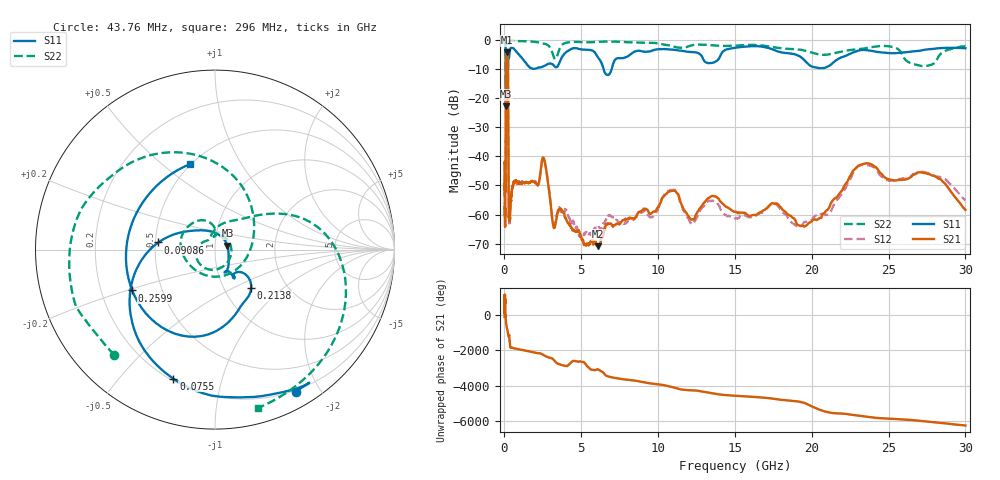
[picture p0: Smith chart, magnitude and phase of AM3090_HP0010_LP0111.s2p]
! Date/Time: Thu, Feb 28, 2019 1:55 PM
! Network Analyzer: Agilent Technologies E8364B Rev: A.07.50.67
! Sweep from 0.010 to 30.000 GHz, 1601 Points, Sweep Type: LOG
! Power Supply: 5.023 V, 0.002 A
# Hz S DB R 50
!freq MagS11 AngS11 MagS21 AngS21 MagS12 AngS12 MagS22 AngS22
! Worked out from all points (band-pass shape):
!   1601 points, 10 MHz to 30 GHz, reference 50 ohm
!   highest |S21| = -4.23 dB at 147.6 MHz (marker M1); lowest = -70.9 dB at 6.08 GHz (marker M2)
!   |S21| within 3 dB of the highest: 101.6 MHz to 216.8 MHz (115.2 MHz wide, 72.4 % of centre)
!   lowest |S11| = -22.8 dB at 99.43 MHz (marker M3), VSWR 1.16, Z = 57.4 + j2.54 ohm
!   |S11| at or under -10 dB: 90.9 MHz to 217.7 MHz (126.8 MHz wide, 82.2 % of centre); 6.451 GHz to 6.979 GHz (528.7 MHz wide, 7.87 % of centre)
!   |S22| runs from -23.8 to -0.2 dB; largest |S21 - S12| = 0.014
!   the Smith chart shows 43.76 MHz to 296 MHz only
!   S11 on the Smith chart (normalised r, x): 43.76 MHz: 0.18, -1.71; 75.5 MHz: 0.21, -0.71; 90.86 MHz: 0.52, +0.05; 213.8 MHz: 1.33, -0.63; 259.9 MHz: 0.34, -0.21; 296 MHz: 0.49, +0.62
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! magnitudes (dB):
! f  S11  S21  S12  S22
! 10 MHz  -0.3  -41.9  -42.1  -0.6
! 38.04 MHz  -0.5  -58.2  -60.9  -1.5
! 43.76 MHz  -0.8  -62.1  -59.4  -1.8
! 47.89 MHz  -0.8  -47.6  -48.9  -1.6
! 75.5 MHz  -2.4  -47.3  -46.9  -4.4
! 90.86 MHz  -9.9  -15.9  -15.8  -16.2
! 99.43 MHz  -22.8  -8.0  -8.0  -14.0
! 144.7 MHz  -15.2  -4.2  -4.2  -21.0
! 147.6 MHz  -15.2  -4.2  -4.2  -20.9
! 213.8 MHz  -10.6  -6.8  -6.7  -18.0
! 259.9 MHz  -5.8  -45.5  -45.2  -1.9
! 296 MHz  -6.1  -60.5  -60.0  -0.8
! 550.5 MHz  -2.8  -50.1  -49.8  -0.3
! 2.084 GHz  -9.8  -49.4  -49.1  -0.7
! 2.558 GHz  -9.0  -40.6  -40.7  -1.3
! 3.188 GHz  -8.6  -63.8  -63.3  -5.6
! 6.08 GHz  -6.0  -70.9  -64.9  -0.7
! 7.926 GHz  -5.9  -61.6  -62.6  -0.8
! 10.86 GHz  -3.3  -52.0  -51.6  -2.0
! 19.8 GHz  -8.4  -62.9  -62.4  -4.1
! 23.48 GHz  -3.4  -42.5  -42.9  -2.9
! 30 GHz  -2.9  -58.4  -55.2  -2.2
